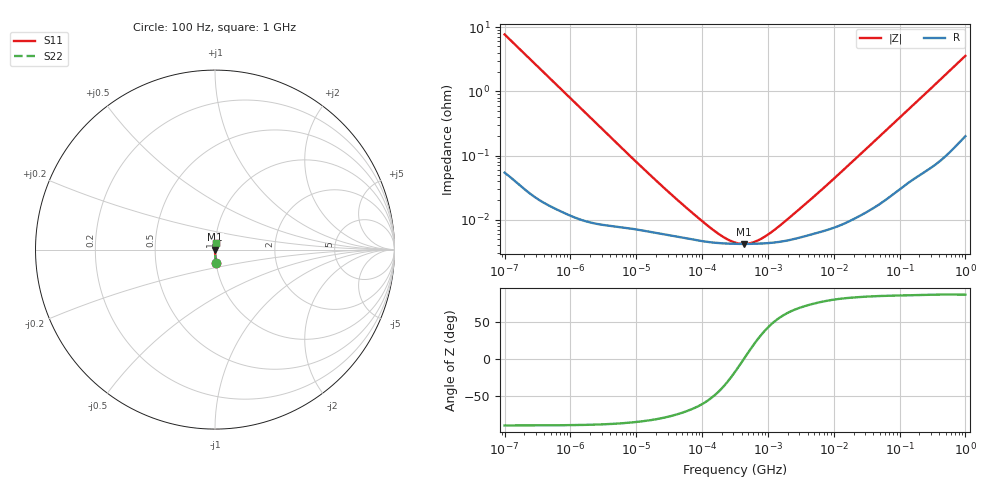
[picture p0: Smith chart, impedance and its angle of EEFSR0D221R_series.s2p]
!  *** S-Parameter ***
!  Copyright (C) Panasonic Industry Corporation
!  Conductive Polymer Aluminum Electrolytic Capacitor (SP-Cap)
!  Parts No. EEFSR0D221R
!  Connection Mode : Series
!  1  o---||---o  2
!  GND o--------o GND
!  Conditions : Temperature = 20 degC , DC Bias = 0 V
! Frequency Range : 100Hz  -  1GHz  [ 401 Steps ]
# Hz S RI R 50
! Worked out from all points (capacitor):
!   401 points, 100 Hz to 1 GHz, reference 50 ohm
!   read as one part in series: C = 207 uF near 108.4 Hz
!   lowest |Z| = 4.19 mohm at 436.5 kHz (marker M1)
!   series resonance near 430.5 kHz, so ESL is about 660 pH
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100  0.00641 -0.0764  0.9936 0.0764  0.9936 0.0764  0.00641 -0.0764
108.3927  0.00552 -0.0706  0.9945 0.0706  0.9945 0.0706  0.00552 -0.0706
175.7924  0.00225 -0.0438  0.9977 0.0438  0.9977 0.0438  0.00225 -0.0438
296.8247  0.000897 -0.026  0.9991 0.026  0.9991 0.026  0.000897 -0.026
1487.647  0.000126 -0.00523  0.9999 0.00523  0.9999 0.00523  0.000126 -0.00523
7161.434  7.55e-05 -0.0011  0.9999 0.0011  0.9999 0.0011  7.55e-05 -0.0011
22130.95  6.11e-05 -0.000365  0.9999 0.000365  0.9999 0.000365  6.11e-05 -0.000365
55911.35  5.16e-05 -0.000149  0.9999 0.000149  0.9999 0.000149  5.16e-05 -0.000149
87096.36  4.74e-05 -9.59e-05  1 9.59e-05  1 9.59e-05  4.74e-05 -9.59e-05
94406.09  4.68e-05 -8.82e-05  1 8.82e-05  1 8.82e-05  4.68e-05 -8.82e-05
102329.3  4.62e-05 -8.1e-05  1 8.1e-05  1 8.1e-05  4.62e-05 -8.1e-05
316227.8  4.2e-05 -1.32e-05  1 1.32e-05  1 1.32e-05  4.2e-05 -1.32e-05
436515.8  4.19e-05 5.92e-07  1 -5.92e-07  1 -5.92e-07  4.19e-05 5.92e-07
1788546  4.65e-05 8.03e-05  1 -8.03e-05  1 -8.03e-05  4.65e-05 8.03e-05
1938653  4.72e-05 8.75e-05  1 -8.75e-05  1 -8.75e-05  4.72e-05 8.75e-05
2187762  4.84e-05 9.92e-05  1 -9.92e-05  1 -9.92e-05  4.84e-05 9.92e-05
4704354  5.93e-05 0.000209  0.9999 -0.000209  0.9999 -0.000209  5.93e-05 0.000209
1.141563e7  7.88e-05 0.000484  0.9999 -0.000484  0.9999 -0.000484  7.88e-05 0.000484
6.99842e7  0.000232 0.00275  0.9998 -0.00275  0.9998 -0.00275  0.000232 0.00275
3.235937e8  0.000821 0.0119  0.9992 -0.0119  0.9992 -0.0119  0.000821 0.0119
9.225714e8  0.00292 0.0329  0.9971 -0.0329  0.9971 -0.0329  0.00292 0.0329
1e9  0.00326 0.0355  0.9967 -0.0355  0.9967 -0.0355  0.00326 0.0355
